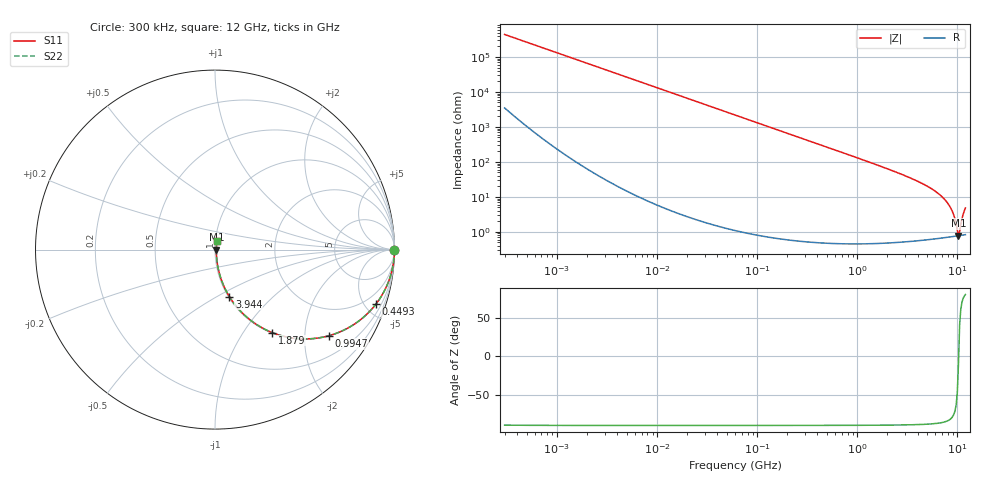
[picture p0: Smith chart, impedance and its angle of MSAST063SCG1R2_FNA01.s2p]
! MSAST063SCG1R2_FNA01  S-PARAMETER MODEL  ( Standard Model )
! Model Generated by TAIYO YUDEN Corporation (http://www.ty-top.com)
! Version 1.0
! TAIYO YUDEN Control No. 241122
! Copyright(c) 2024 TAIYO YUDEN CO.,LTD. All Rights Reserved.
! Product Description (link to TY-COMPAS)
! https://ds.yuden.co.jp/TYCOMPAS/or/detail?pn=MSAST063SCG1R2CFNA01&u=M
! Products Name : Multilayer Ceramic Capacitors
! Characteristics :
!  Capacitance : 1.2 [pF] , Rated Voltage : 25 [V] , TCC : CG / C0G
!  Case Size : 0.6 x 0.3 / 0.024 x 0.012 [mm/inch] , Thickness : 0.3 / 0.012 [mm/inch]
!  (Conditions: Temperature = 25 [degC] , DC Bias Voltage = 0 [V])
! External Node Assignments :
!  1  o---| |---o  2
! GND o---------o GND
! Frequency Range : 0.3MHz  -  12000MHz  [ 401 STEP ]
# MHZ S RI R 50
! Freq[MHz].  S11 Real  S11 Imag  S21 Real  S21 Imag  S12 Real  S12 Imag  S22 Real  S22 Imag
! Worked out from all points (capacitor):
!   401 points, 300 kHz to 12 GHz, reference 50 ohm
!   read as one part in series: C = 1.21 pF near 316.3 kHz
!   lowest |Z| = 788 mohm at 10.24 GHz (marker M1)
!   series resonance near 10.28 GHz, so ESL is about 200 pH
!   S11 on the Smith chart (normalised r, x): 300 kHz: open; 449.3 MHz: 1.01, -5.87; 994.7 MHz: 1.01, -2.63; 1.879 GHz: 1.01, -1.36; 3.944 GHz: 1.01, -0.57; 12 GHz: 1.02, +0.09
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0.3  1 -0.000227  1.85e-06 0.000227  1.85e-06 0.000227  1 -0.000227
1.769972  1 -0.00134  3.2e-06 0.00134  3.2e-06 0.00134  1 -0.00134
10.44266  0.9999 -0.00791  6.6e-05 0.00791  6.6e-05 0.00791  0.9999 -0.00791
60  0.9979 -0.0453  0.00208 0.0453  0.00208 0.0453  0.9979 -0.0453
159.8975  0.9855 -0.1193  0.0145 0.1193  0.0145 0.1193  0.9855 -0.1193
353.9943  0.9325 -0.2501  0.0675 0.2501  0.0675 0.2501  0.9325 -0.2501
449.3064  0.8955 -0.3051  0.1045 0.3051  0.1045 0.3051  0.8955 -0.3051
668.5285  0.7941 -0.4032  0.2059 0.4032  0.2059 0.4032  0.7941 -0.4032
994.7115  0.6333 -0.4802  0.3667 0.4802  0.3667 0.4802  0.6333 -0.4802
1878.541  0.3172 -0.4619  0.6828 0.4619  0.6828 0.4619  0.3172 -0.4619
2088.533  0.2705 -0.4402  0.7295 0.4402  0.7295 0.4402  0.2705 -0.4402
3944.255  0.0798 -0.2614  0.9202 0.2614  0.9202 0.2614  0.0798 -0.2614
5715.274  0.0306 -0.154  0.9694 0.154  0.9694 0.154  0.0306 -0.154
7448.838  0.0137 -0.0827  0.9863 0.0827  0.9863 0.0827  0.0137 -0.0827
8732.115  0.00897 -0.0417  0.991 0.0417  0.991 0.0417  0.00897 -0.0417
9207.246  0.00818 -0.0282  0.9918 0.0282  0.9918 0.0282  0.00818 -0.0282
9968.853  0.00769 -0.00802  0.9923 0.00802  0.9923 0.00802  0.00769 -0.00802
10236.47  0.00771 -0.00128  0.9923 0.00128  0.9923 0.00128  0.00771 -0.00128
10511.28  0.00784 0.00662  0.9922 -0.00662  0.9922 -0.00662  0.00784 0.00662
10793.46  0.00808 0.0139  0.9919 -0.0139  0.9919 -0.0139  0.00808 0.0139
11380.75  0.00896 0.0297  0.991 -0.0297  0.991 -0.0297  0.00896 0.0297
12000  0.0105 0.0465  0.9895 -0.0465  0.9895 -0.0465  0.0105 0.0465
